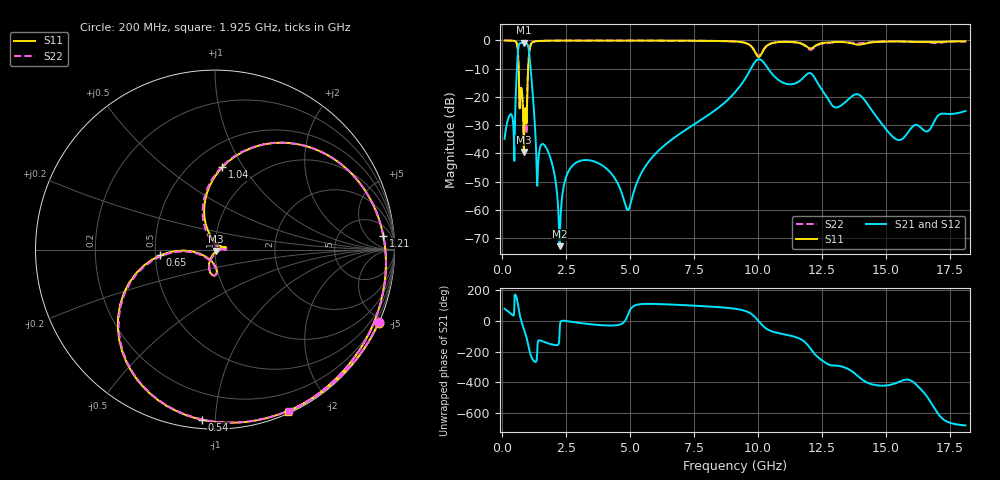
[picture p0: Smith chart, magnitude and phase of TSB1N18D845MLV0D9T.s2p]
! TSB1N18D845MLV0D9T  S-PARAMETER MODEL  ( General Type )
! Model Generated by TAIYO YUDEN Corporation (https://www.yuden.co.jp/en/)
! Version 1.0
! TAIYO YUDEN Control No. 20190830
! Copyright(c) 2019 TAIYO YUDEN CO.,LTD. All Rights Reserved.
! Products Name : Multilayer Ceramic Devices
! Characteristics :
!  Passband freq : 729-960MHz ( At Passband , Insertion Loss : 2.0dB , VSWR 2.0 ),
!  Attenuation : 17dB min at 240 to 480MHz, 15dB min at 1458 to 6720MHz , Impedance : 50 Ohm ,
!  Case Size : 1.6 x 0.8 / 0.063 x 0.031 [mm/inch] , Thickness : 0.65 / 0.026 [mm/inch]
!  (Conditions: Temperature = 25 degC , DC Bias Current/Voltage = 0A / 0V)
! External Node Assignments :
!  1  o---|-------|---o  2
!  |  BPF  |
! GND o---|-------|---o GND
! Frequency Range : 100MHz  -  18.1GHz  [ 3601 STEP ]
# MHZ S RI R 50
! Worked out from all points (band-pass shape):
!   3601 points, 100 MHz to 18.1 GHz, reference 50 ohm
!   highest |S21| = -0.77 dB at 840 MHz (marker M1); lowest = -72.9 dB at 2.245 GHz (marker M2)
!   |S21| within 3 dB of the highest: 624.6 MHz to 1.051 GHz (426 MHz wide, 50.9 % of centre)
!   lowest |S11| = -39.5 dB at 850 MHz (marker M3), VSWR 1.02, Z = 50.7 - j0.821 ohm
!   |S11| at or under -10 dB: 649 MHz to 1.02 GHz (370.6 MHz wide, 44.4 % of centre)
!   |S22| runs from -35.1 to 0.0 dB; largest |S21 - S12| = 8.8e-06
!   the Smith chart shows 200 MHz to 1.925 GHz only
!   S11 on the Smith chart (normalised r, x): 200 MHz: 0.02, -4.69; 540 MHz: 0.05, -0.93; 650 MHz: 0.53, -0.04; 1.04 GHz: 0.70, +0.81; 1.21 GHz: 11, +16; 1.925 GHz: 0.02, -1.55
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100  0.9787 -0.2034  0.0037 0.0177  0.0037 0.0177  0.9788 -0.2025
200  0.9117 -0.407  0.0143 0.032  0.0143 0.032  0.9125 -0.4053
540  -0.0719 -0.9482  -0.1145 0.033  -0.1145 0.033  -0.0647 -0.9481
650  -0.3047 -0.0319  0.2183 0.7719  0.2183 0.7719  -0.3018 -0.0362
750  -0.00887 -0.1442  0.9023 0.000855  0.9023 0.00086  -0.0105 -0.1437
840  -0.00519 -0.0199  0.6256 -0.6675  0.6256 -0.6675  0.00211 -0.0211
850  0.00675 -0.0081  0.564 -0.7199  0.564 -0.7199  0.0144 -0.0108
1040  0.0408 0.4592  -0.6882 -0.1242  -0.6882 -0.1242  0.037 0.461
1210  0.9374 0.0782  -0.0267 0.0921  -0.0267 0.0921  0.9366 0.0858
1390  0.88 -0.4194  -0.00339 -0.00228  -0.00339 -0.00229  0.8828 -0.4145
1925  0.4076 -0.9029  -0.00651 -0.00338  -0.00651 -0.00338  0.4123 -0.9008
2245  0.1672 -0.9787  2.78e-06 -0.000227  2.83e-06 -0.000227  0.1722 -0.9779
2540  -0.019 -0.9937  0.00423 -0.000145  0.00423 -0.000145  -0.014 -0.9939
3100  -0.2935 -0.9502  0.0072 -0.002  0.0072 -0.002  -0.289 -0.9518
4915  -0.7538 -0.6482  0.000779 0.000613  0.000779 0.000613  -0.7512 -0.6511
6100  -0.8823 -0.4552  -0.00355 0.0104  -0.00355 0.0104  -0.8806 -0.4583
9100  -0.9581 0.0238  0.0244 0.1186  0.0244 0.1186  -0.9587 0.0173
10030  -0.5098 -0.00964  0.4643 -0.032  0.4643 -0.032  -0.5311 -0.0181
10850  -0.9358 -0.0577  0.0262 -0.1903  0.0262 -0.1903  -0.936 -0.044
12100  -0.7275 0.0276  -0.2477 0.0544  -0.2477 0.0544  -0.6892 0.0221
15100  -0.9138 0.2892  0.0125 -0.02  0.0125 -0.02  -0.9115 0.3075
18100  -0.763 0.5857  0.0429 0.0365  0.0429 0.0365  -0.7501 0.5878
